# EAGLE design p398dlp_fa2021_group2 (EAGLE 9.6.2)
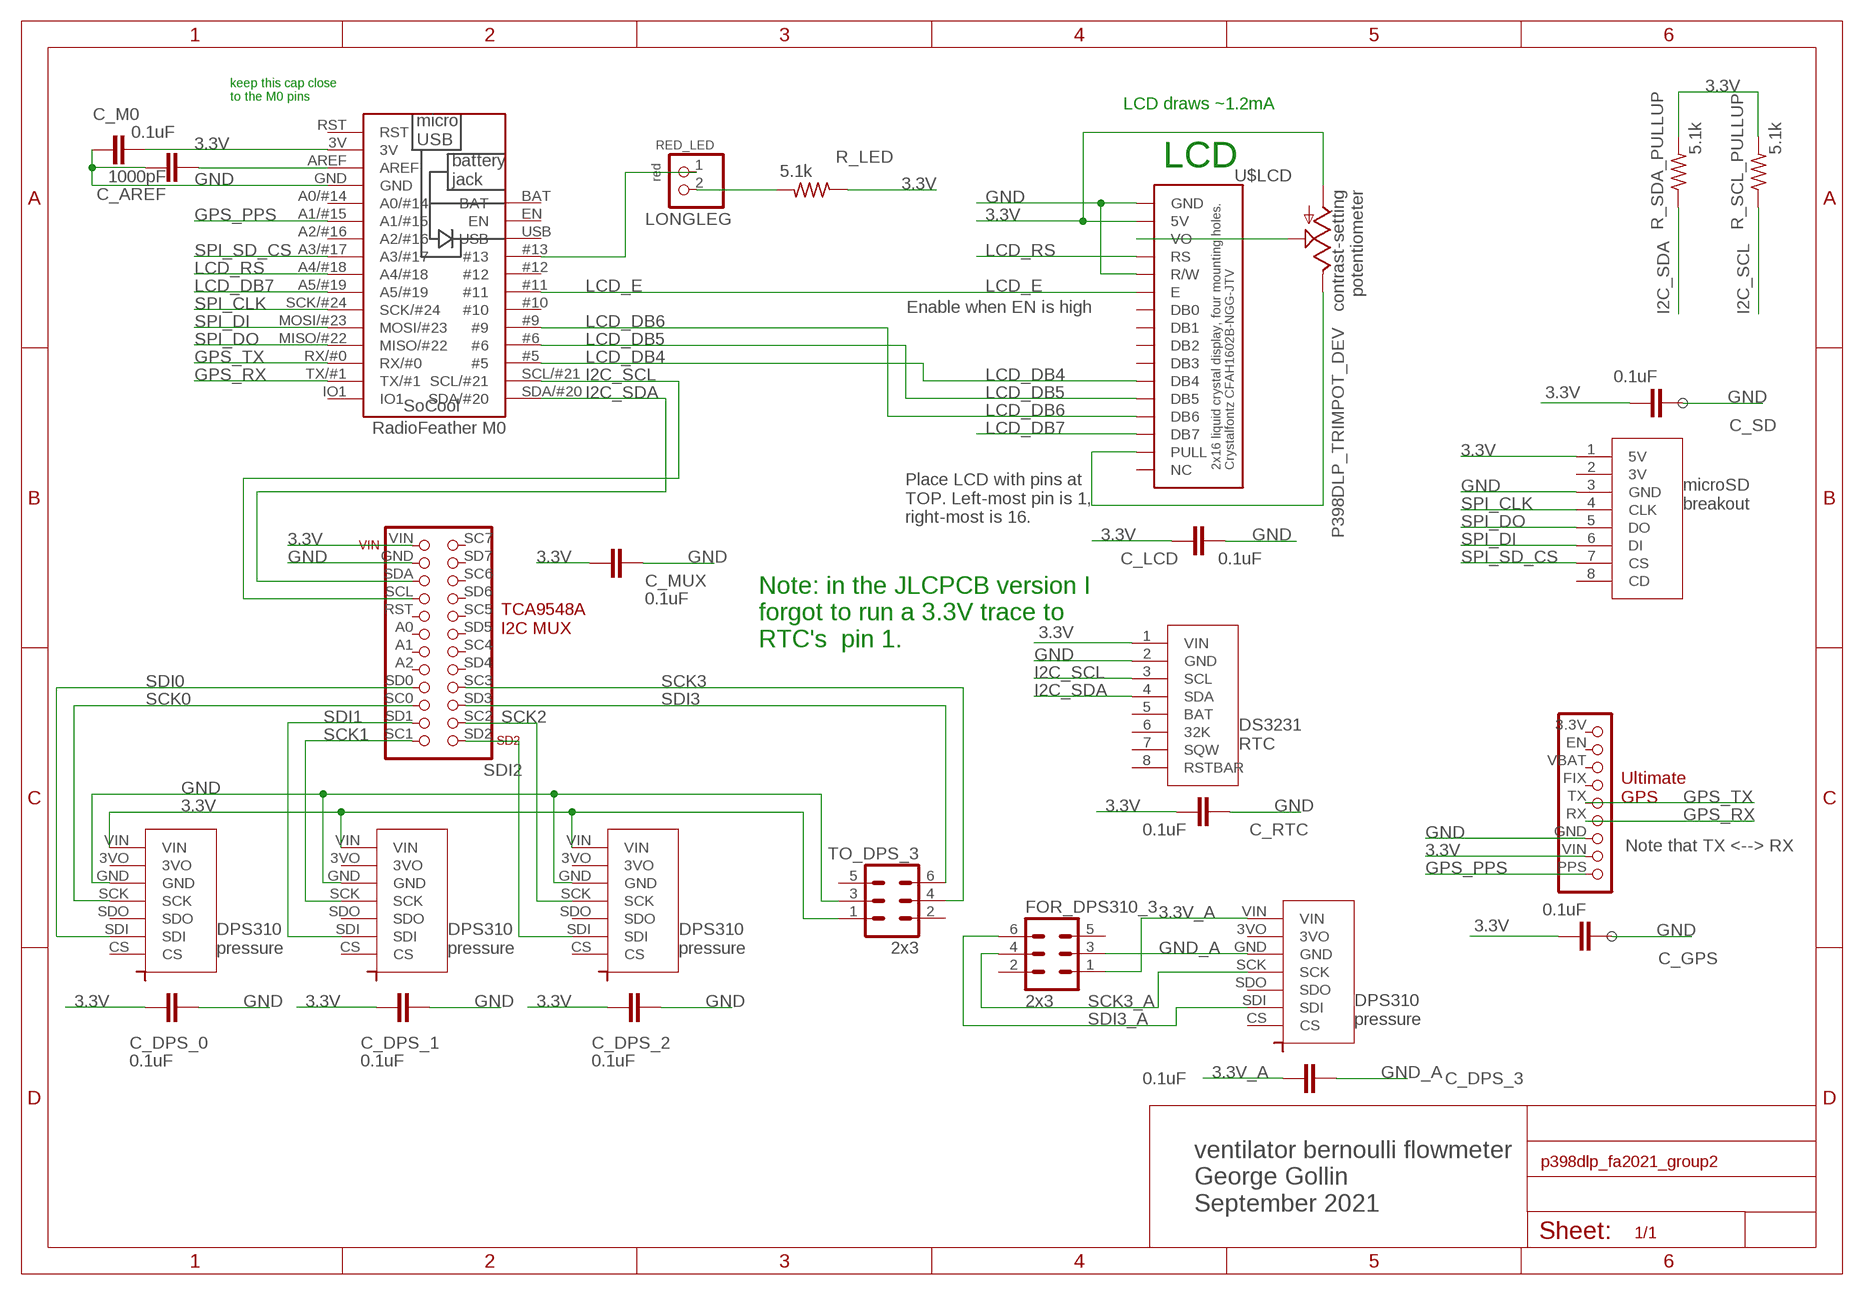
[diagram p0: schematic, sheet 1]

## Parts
C_AREF  1000pF  C5/3.5  [C5B3.5]
C_DPS_0  0.1uF  C5/3.5  [C5B3.5]
C_DPS_1  0.1uF  C5/3.5  [C5B3.5]
C_DPS_2  0.1uF  C5/3.5  [C5B3.5]
C_DPS_3  0.1uF  C5/3.5  [C5B3.5]
C_GPS  0.1uF  C5/3.5  [C5B3.5]
C_LCD  0.1uF  C5/3.5  [C5B3.5]
C_M0  0.1uF  C5/3.5  [C5B3.5]
C_MUX  0.1uF  C5/3.5  [C5B3.5]
C_RTC  0.1uF  C5/3.5  [C5B3.5]
C_SD  0.1uF  C5/3.5  [C5B3.5]
DPS310_0  P398DLP_DPS310_DEV  [P398DLP_DPS310_PKG]
DPS310_1  P398DLP_DPS310_DEV  [P398DLP_DPS310_PKG]
DPS310_2  P398DLP_DPS310_DEV  [P398DLP_DPS310_PKG]
DPS310_3  P398DLP_DPS310_DEV  [P398DLP_DPS310_PKG]
FOR_DPS310_3  2x3  P398DLP_RIBBON_PCB_2X3_DEV  [06V]
R_LED  5.1k  R-US_0207/7  [0207/7]
R_SCL_PULLUP  5.1k  R-US_0207/7  [0207/7]
R_SDA_PULLUP  5.1k  R-US_0207/7  [0207/7]
RED_LED  red  PINHD-1X2  [1X02]
TO_DPS_3  2x3  P398DLP_RIBBON_PCB_2X3_DEV  [06V]
U$5  P398DLP_TCA9548A_MUX_DEV  [P398DLP_TCA9548A_MUX_PKG]
U$6  P398DLP_DS3231_DEV  [P398DLP_DS3231_PKG]
U$19  P398DLP_TRIMPOT_DEV  [P398DLP_TRIMPOT_PKG]
U$GPS1  P398DLP_ULTIMATE_GPS_DEV  [P398DLP_ULTIMATE_GPS_PKG]
U$LCD  P398DLP_LCD_16X2_DEV  [P398DLP_LCD_16X2_PKG]
U$MICROSD1  P398DLP_MICROSD_DEV  [P398DLP_MICROSD_PKG]
U$RADIOFEATHER  P398DLP_RADIOFEATHER_MO_DEV  [P398DLP_RADIOFEATHER_M0_PKG]

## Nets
3.3V [power]: C_DPS_0.2 C_DPS_1.2 C_DPS_2.2 C_GPS.2 C_LCD.2 C_M0.1 C_MUX.2 C_RTC.2 C_SD.2 DPS310_0.VIN DPS310_1.VIN DPS310_2.VIN R_LED.1 R_SCL_PULLUP.2 R_SDA_PULLUP.2 TO_DPS_3.1 U$5.VIN U$6.1(VIN) U$19.BOTTOM U$GPS1.VIN U$LCD.5V U$MICROSD1.1(5V) U$RADIOFEATHER.3V
3.3V_A: C_DPS_3.2 DPS310_3.VIN FOR_DPS310_3.1
GND [power]: C_AREF.2 C_DPS_0.1 C_DPS_1.1 C_DPS_2.1 C_GPS.1 C_LCD.1 C_M0.2 C_MUX.1 C_RTC.1 C_SD.1 DPS310_0.GND DPS310_1.GND DPS310_2.GND TO_DPS_3.3 U$5.GND U$6.2(GND) U$GPS1.GND U$LCD.GND U$LCD.R/W U$MICROSD1.3(GND) U$RADIOFEATHER.GND
GND_A: C_DPS_3.1 DPS310_3.GND FOR_DPS310_3.3
GPS_PPS: U$GPS1.PPS U$RADIOFEATHER.A1/#15
GPS_RX: U$GPS1.RX U$RADIOFEATHER.TX/#1
GPS_TX: U$GPS1.TX U$RADIOFEATHER.RX/#0
I2C_SCL: R_SCL_PULLUP.1 U$5.SCL U$6.3(SCL) U$RADIOFEATHER.SCL/#21
I2C_SDA: R_SDA_PULLUP.1 U$5.SDA U$6.4(SDA) U$RADIOFEATHER.SDA/#20
LCD_DB4: U$LCD.DB4 U$RADIOFEATHER.#5
LCD_DB5: U$LCD.DB5 U$RADIOFEATHER.#6
LCD_DB6: U$LCD.DB6 U$RADIOFEATHER.#9
LCD_DB7: U$LCD.DB7 U$RADIOFEATHER.A5/#19
LCD_E: U$LCD.E U$RADIOFEATHER.#11
LCD_RS: U$LCD.RS U$RADIOFEATHER.A4/#18
LONGLEG: R_LED.2 RED_LED.2
N$1: U$19.TOP U$LCD.PULL
N$5: C_AREF.1 U$RADIOFEATHER.AREF
N$6: U$19.TAP U$LCD.VO
SCK0: DPS310_0.SCK U$5.SC0
SCK1: DPS310_1.SCK U$5.SC1
SCK2: DPS310_2.SCK U$5.SC2
SCK3: TO_DPS_3.4 U$5.SC3
SCK3_A: DPS310_3.SCK FOR_DPS310_3.4
SDI0: DPS310_0.SDI U$5.SD0
SDI1: DPS310_1.SDI U$5.SD1
SDI2: DPS310_2.SDI U$5.SD2
SDI3: TO_DPS_3.6 U$5.SD3
SDI3_A: DPS310_3.SDI FOR_DPS310_3.6
SPI_CLK: U$MICROSD1.4(CLK) U$RADIOFEATHER.SCK/#24
SPI_DI: U$MICROSD1.6(DI) U$RADIOFEATHER.MOSI/#23
SPI_DO: U$MICROSD1.5(DO) U$RADIOFEATHER.MISO/#22
SPI_SD_CS: U$MICROSD1.7(CS) U$RADIOFEATHER.A3/#17
WATCHDOG_PULSE: RED_LED.1 U$RADIOFEATHER.#13
Unconnected: DPS310_0.3VO DPS310_0.CS DPS310_0.SDO DPS310_1.3VO DPS310_1.CS DPS310_1.SDO DPS310_2.3VO DPS310_2.CS DPS310_2.SDO DPS310_3.3VO DPS310_3.CS DPS310_3.SDO FOR_DPS310_3.2 FOR_DPS310_3.5 TO_DPS_3.2 TO_DPS_3.5 U$5.A0 U$5.A1 U$5.A2 U$5.RST U$5.SC4 U$5.SC5 U$5.SC6 U$5.SC7 U$5.SD4 U$5.SD5 U$5.SD6 U$5.SD7 U$6.5(BAT) U$6.6(32K) U$6.7(SQW) U$6.8(RSTBAR) U$GPS1.3.3V U$GPS1.EN U$GPS1.FIX U$GPS1.VBAT U$LCD.DB0 U$LCD.DB1 U$LCD.DB2 U$LCD.DB3 U$LCD.NC U$MICROSD1.2(3V) U$MICROSD1.8(CD) U$RADIOFEATHER.#10 U$RADIOFEATHER.#12 U$RADIOFEATHER.A0/#14 U$RADIOFEATHER.A2/#16 U$RADIOFEATHER.BAT U$RADIOFEATHER.EN U$RADIOFEATHER.IO1 U$RADIOFEATHER.RST U$RADIOFEATHER.USB

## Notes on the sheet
- keep this cap close 
  to the M0 pins
- LCD draws ~1.2mA
- LCD
- contrast-setting
  potentiometer
- Enable when EN is high
- Place LCD with pins at 
  TOP. Left-most pin is 1, 
  right-most is 16.
- Note: in the JLCPCB version I
  forgot to run a 3.3V trace to
  RTC's  pin 1.
- Note that TX <--> RX
- ventilator bernoulli flowmeter
  George Gollin
  September 2021

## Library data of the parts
C_AREF C_DPS_0 C_DPS_1-C_DPS_3 C_GPS C_LCD C_M0 C_MUX C_RTC C_SD = capacitor-wima:C: CAPACITOR
DPS310_0 DPS310_1-DPS310_3 = p398dlp:P398DLP_DPS310_DEV: DPS310 precision pressure and temperature sensor. Adafruit 4494
FOR_DPS310_3 TO_DPS_3 = p398dlp:P398DLP_RIBBON_PCB_2X3_DEV: CONNECTOR; OC_FARNELL: unknown; OC_NEWARK: unknown
R_LED R_SCL_PULLUP R_SDA_PULLUP = resistor:R-US_: RESISTOR, American symbol
RED_LED = p398dlp_sp2020:PINHD-1X2: PIN HEADER
U$5 = p398dlp:P398DLP_TCA9548A_MUX_DEV: TCA9548A I2C MUX
U$6 = p398dlp:P398DLP_DS3231_DEV: DS3231 real time clock with battery backup
U$19 = p398dlp:P398DLP_TRIMPOT_DEV: trimpot
U$GPS1 = p398dlp:P398DLP_ULTIMATE_GPS_DEV: Adafruit "ultimate GPS" breakout board
U$LCD = p398dlp:P398DLP_LCD_16X2_DEV: 2x16 liquid crystal display, four mounting holes. Crystalfontz CFAH1602B-NGG-JTV
U$MICROSD1 = p398dlp:P398DLP_MICROSD_DEV: Adafruit microSD reader breakout board
U$RADIOFEATHER = p398dlp:P398DLP_RADIOFEATHER_MO_DEV: Adafruit RadioFeather M0 processor

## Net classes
1 power: width 0.305 mm

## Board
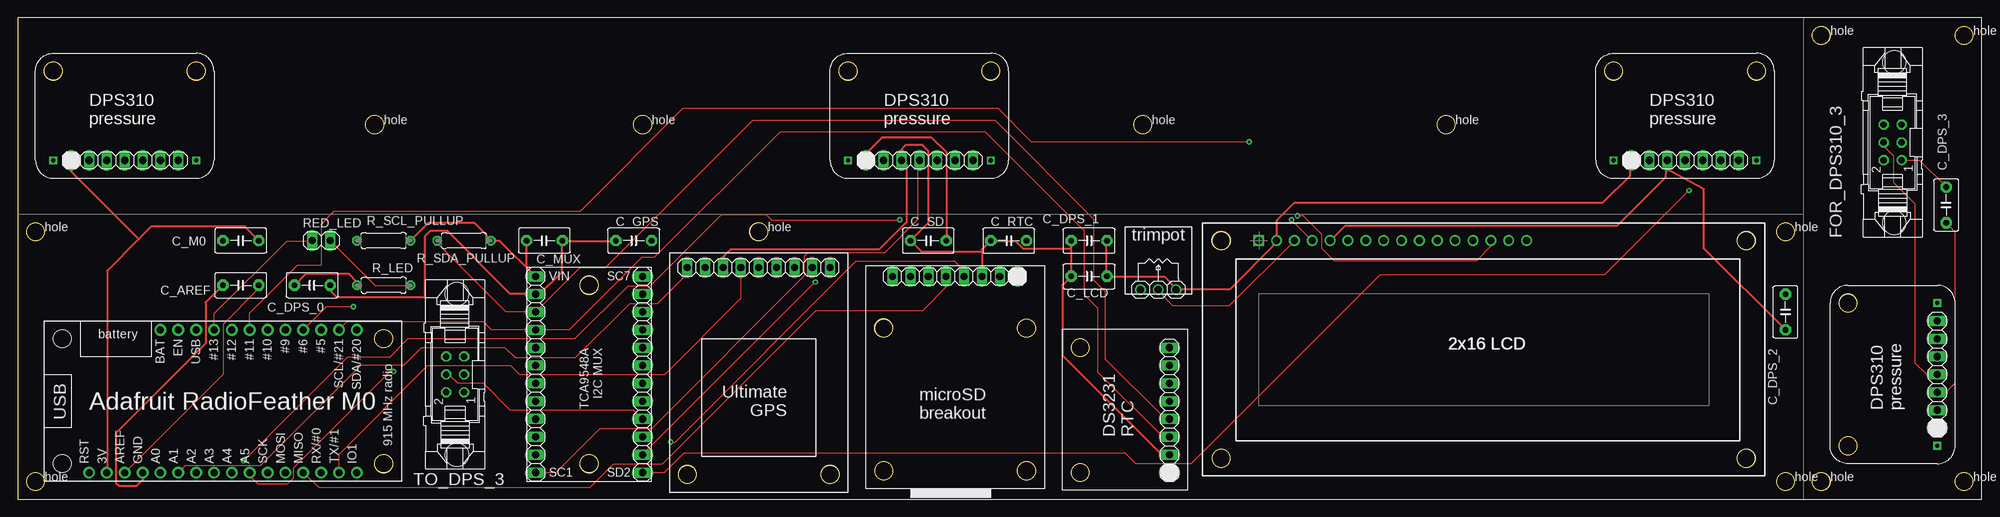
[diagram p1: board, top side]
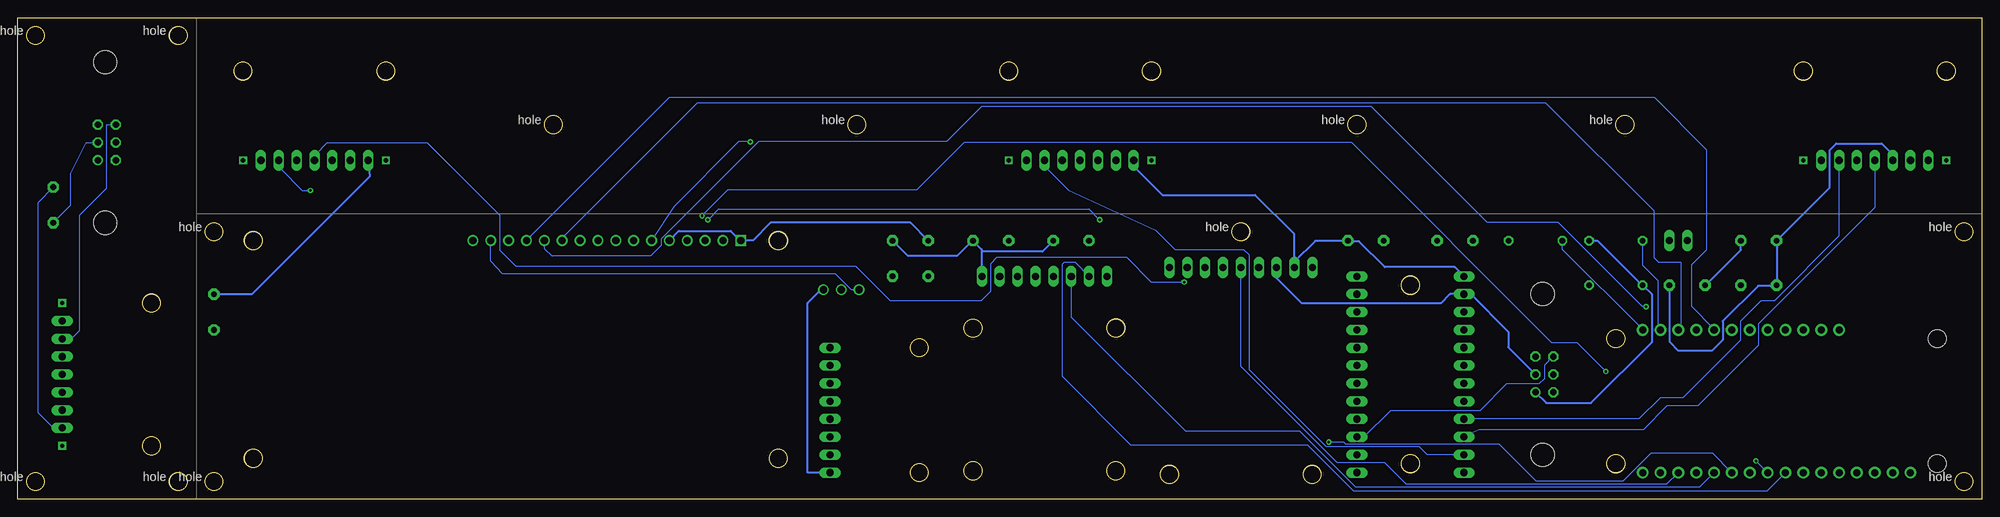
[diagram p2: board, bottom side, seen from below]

Size 279.4 x 68.58 mm. Coordinates in mm from the lower left corner, seen from the top.
Outline: 0,0 279.4,0 279.4,68.58 0,68.58 0,0
Copper layers (1*16): Top 0.035mm / dielectric 1.5mm / Bottom 0.035mm
Design rules "default": minimum track width 6mil, minimum drill 0.35mm, track to track 6mil, track to pad 6mil, pad to pad 6mil, via to via 6mil, smd to smd 6mil, copper to edge 40mil, drill to drill 6mil, minimum pad ring 10mil, minimum via ring 8mil, stop-mask expansion 4mil, vias tented up to drill 0mil, thermal gap 10mil

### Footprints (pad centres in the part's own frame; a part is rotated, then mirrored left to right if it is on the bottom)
C5B3.5 = drill 0.813 pad 1.6 octagon: 1 -2.54,0; 2 2.54,0
P398DLP_DPS310_PKG = drill 1.016 long: 3VO 7.62,2.54; CS 20.32,2.54; GND 10.16,2.54; SCK 12.7,2.54; SDI 17.78,2.54; SDO 15.24,2.54; VIN 5.08,2.54 | drill 0.6 square: P$1 2.54,2.54; P$2 22.86,2.54 | hole 2.54: 22.86,15.24; 2.54,15.24
06V = drill 0.914: 1 -2.54,-1.27 | drill 0.914 octagon: 2 -2.54,1.27; 3 0,-1.27; 4 0,1.27; 5 2.54,-1.27; 6 2.54,1.27 | hole 3.302: 11.43,-0.254; -11.43,-0.254
0207/7 = drill 0.813 octagon: 1 -3.81,0; 2 3.81,0
1X02 = drill 1.016 long: 1 -1.27,0; 2 1.27,0
P398DLP_MOUNTING_HOLE_PKG = hole 2.54: 0,0
P398DLP_TCA9548A_MUX_PKG = drill 1.016 long: A0 12.7,0; A1 15.24,0; A2 17.78,0; GND 2.54,0; RST 10.16,0; SC0 22.86,0; SC1 27.94,0; SC2 25.4,15.24; SC3 20.32,15.24; SC4 15.24,15.24; SC5 10.16,15.24; SC6 5.08,15.24; SC7 0,15.24; SCL 7.62,0; SD0 20.32,0; SD1 25.4,0; SD2 27.94,15.24; SD3 22.86,15.24; SD4 17.78,15.24; SD5 12.7,15.24; SD6 7.62,15.24; SD7 2.54,15.24; SDA 5.08,0; VIN 0,0 | hole 2.54: 1.27,7.62; 26.67,7.62
P398DLP_DS3231_PKG = drill 1.016 long: 1 0,0; 2 2.54,0; 3 5.08,0; 4 7.62,0; 5 10.16,0; 6 12.7,0; 7 15.24,0; 8 17.78,0 | hole 2.54: 0,12.7; 17.78,12.7
P398DLP_TRIMPOT_PKG = drill 1.016: BOTTOM 7.303,0.635; TAP 4.763,0.635; TOP 2.223,0.635
P398DLP_ULTIMATE_GPS_PKG = drill 1.016 long: 3.3V 0,0; EN 2.54,0; FIX 7.62,0; GND 15.24,0; PPS 20.32,0; RX 12.7,0; TX 10.16,0; VBAT 5.08,0; VIN 17.78,0 | hole 2.54: 0,29.464; 20.32,29.464
P398DLP_LCD_16X2_PKG = drill 1.016: 5V 2.544,0.006; DB0 15.244,0.006; DB1 17.784,0.006; DB2 20.324,0.006; DB3 22.864,0.006; DB4 25.404,0.006; DB5 27.944,0.006; DB6 30.484,0.006; DB7 33.024,0.006; E 12.704,0.006; NC 38.104,0.006; PULL 35.564,0.006; R/W 10.164,0.006; RS 7.624,0.006; VO 5.084,0.006 | drill 1.016 square: GND 0.004,0.006 | hole 2.54: -5.334,0; -5.334,-30.988; 69.342,-30.988; 69.342,0
P398DLP_MICROSD_PKG = drill 1.016 long: 1 0,0; 2 2.54,0; 3 5.08,0; 4 7.62,0; 5 10.16,0; 6 12.7,0; 7 15.24,0; 8 17.78,0 | hole 2.54: -1.27,27.686; 19.05,27.686; 19.05,7.366; -1.27,7.366
P398DLP_RADIOFEATHER_M0_PKG = drill 1 pad 1.676: 3V 8.89,1.27; #5 39.37,21.59; #6 36.83,21.59; #9 34.29,21.59; #10 31.75,21.59; #11 29.21,21.59; #12 26.67,21.59; #13 24.13,21.59; A0/#14 16.51,1.27; A1/#15 19.05,1.27; A2/#16 21.59,1.27; A3/#17 24.13,1.27; A4/#18 26.67,1.27; A5/#19 29.21,1.27; AREF 11.43,1.27; BAT 16.51,21.59; EN 19.05,21.59; GND 13.97,1.27; IO1 44.45,1.27; MISO/#22 36.83,1.27; MOSI/#23 34.29,1.27; RST 6.35,1.27; RX/#0 39.37,1.27; SCK/#24 31.75,1.27; SCL/#21 41.91,21.59; SDA/#20 44.45,21.59; TX/#1 41.91,1.27; USB 21.59,21.59 | hole 2.54: 48.26,2.54; 48.26,20.32; 2.54,20.32; 2.54,2.54

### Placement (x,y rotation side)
C_AREF  31.75,30.48 180 top
C_DPS_0  41.91,30.48 180 top
C_DPS_1  152.4,36.83 0 top
C_DPS_2  251.46,26.67 90 top
C_DPS_3  274.32,41.91 90 top
C_GPS  87.63,36.83 0 top
C_LCD  152.4,31.75 0 top
C_M0  31.75,36.83 180 top
C_MUX  74.93,36.83 180 top
C_RTC  140.97,36.83 0 top
C_SD  129.54,36.83 0 top
DPS310_0  2.54,45.72 0 top
DPS310_1  115.57,45.72 0 top
DPS310_2  224.47,45.72 0 top
DPS310_3  275.59,5.08 90 top
FOR_DPS310_3  266.7,50.8 90 top
R_LED  52.07,30.48 0 top
R_SCL_PULLUP  52.07,36.83 0 top
R_SDA_PULLUP  63.5,36.83 0 top
RED_LED  43.18,36.83 0 top
TO_DPS_3  62.23,17.78 90 top
U$1  [P398DLP_MOUNTING_HOLE_PKG]  2.54,2.54 0 top
U$2  [P398DLP_MOUNTING_HOLE_PKG]  2.54,38.1 0 top
U$3  [P398DLP_MOUNTING_HOLE_PKG]  105.41,38.1 0 top
U$4  [P398DLP_MOUNTING_HOLE_PKG]  251.46,2.54 0 top
U$5  73.66,31.75 270 top
U$6  163.83,3.81 90 top
U$7  [P398DLP_MOUNTING_HOLE_PKG]  251.46,38.1 0 top
U$8  [P398DLP_MOUNTING_HOLE_PKG]  256.54,66.04 0 top
U$9  [P398DLP_MOUNTING_HOLE_PKG]  276.86,66.04 0 top
U$10  [P398DLP_MOUNTING_HOLE_PKG]  256.54,2.54 0 top
U$11  [P398DLP_MOUNTING_HOLE_PKG]  276.86,2.54 0 top
U$12  [P398DLP_MOUNTING_HOLE_PKG]  50.8,53.34 0 top
U$13  [P398DLP_MOUNTING_HOLE_PKG]  88.9,53.34 0 top
U$14  [P398DLP_MOUNTING_HOLE_PKG]  160.02,53.34 0 top
U$15  [P398DLP_MOUNTING_HOLE_PKG]  203.2,53.34 0 top
U$19  157.48,29.21 0 top
U$GPS1  115.57,33.02 180 top
U$LCD  176.53,36.83 0 top
U$MICROSD1  142.24,31.75 180 top
U$RADIOFEATHER  3.81,2.54 0 top

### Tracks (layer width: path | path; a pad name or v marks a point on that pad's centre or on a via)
3.3V
  Top 0.305: DPS310_0.VIN 7.62,46.69 17.25,37.06 | C_M0.1 34.29,36.88 32.33,38.84 19.02,38.84 17.25,37.06 | 17.25,37.06 12.72,32.54 12.72,3.81 U$RADIOFEATHER.3V | R_LED.1 48.26,30.94 47.07,32.13 41.05,32.13 39.4,30.48 C_DPS_0.2 | R_SCL_PULLUP.2 58.45,39.4 64.92,39.4 67.31,37.01 R_SDA_PULLUP.2 67.36,36.8 68.58,36.8 73.61,31.77 U$5.VIN 72.39,33.02 C_MUX.2 | C_DPS_1.2 154.91,36.8 154.91,31.85 C_LCD.2 154.99,31.7 163.09,31.7 164.78,30.01 U$19.BOTTOM 164.9,29.95 172.49,29.95 179.07,36.53 U$LCD.5V 179.15,36.96 179.15,39.73 181.63,42.22 225.48,42.22 229.36,46.1 229.36,48.23 DPS310_2.VIN | DPS310_1.VIN 120.4,48.9 122.99,51.49 130.02,51.49 132.1,49.4 132.1,36.85 C_SD.2
  Bottom 0.305: R_SCL_PULLUP.2 55.85,36.8 54.63,36.8 48.31,30.48 R_LED.1 48.16,30.4 46.97,29.21 46.97,22.35 55.6,13.72 61.98,13.72 TO_DPS_3.1 | U$5.VIN 74.98,33.07 84.94,33.07 88.59,36.73 90.07,36.73 C_GPS.2 90.22,36.8 94.82,36.8 97.79,33.83 U$GPS1.VIN 97.79,37.74 103.38,43.33 116.56,43.33 120.4,47.17 120.4,48.23 DPS310_1.VIN | C_M0.1 34.29,35.51 39.32,30.48 C_DPS_0.2 | DPS310_2.VIN 229.34,45.95 246.02,29.26 251.46,29.26 C_DPS_2.2 | 142.26,35.28 142.26,35.59 C_RTC.2 143.64,36.8 145.8,34.65 152.76,34.65 C_DPS_1.2 | 142.26,35.28 142.26,31.77 U$MICROSD1.1 | 142.26,35.28 133.66,35.28 132.13,36.8 C_SD.2 | U$6.1 167,3.81 167,27.94 165.1,29.84 U$19.BOTTOM
3.3V_A
  Top 0.152: FOR_DPS310_3.1 268,48.23 270.59,48.23 274.32,44.5 C_DPS_3.2
  Bottom 0.152: DPS310_3.VIN 274.32,10.16 276.56,12.39 276.56,42.19 274.32,44.42 C_DPS_3.2
GND
  Top 0.305: U$RADIOFEATHER.GND 17.78,2.77 16.92,1.91 14.45,1.91 13.97,2.39 13.97,9.42 26.75,22.2 26.75,28.04 29.18,30.48 C_AREF.2 | 77.42,36.8 77.42,32.36 74.27,29.21 U$5.GND 73.53,29.26 70.05,29.26 61.14,38.18 58.65,38.18 57.91,37.44 57.91,28.8 57.84,28.73 45.47,28.73 44.45,29.74 C_DPS_0.1 | 77.42,36.8 77.42,36.83 C_MUX.1 | 77.42,36.8 85.04,36.8 C_GPS.1 | C_DPS_2.1 251.46,24.16 239.88,35.74 239.88,44.17 234.42,47.1 DPS310_2.GND 234.42,45.85 227.53,38.96 188.85,38.96 186.77,36.88 U$LCD.R/W | 137.16,35.28 137.16,35.59 138.38,36.8 C_RTC.1 138.53,36.73 142.04,36.73 143.1,35.66 149.88,35.66 | 137.16,35.28 U$MICROSD1.3 | 127.03,36.88 129.54,39.4 129.54,49.58 128.73,50.39 126.29,50.39 125.48,49.59 DPS310_1.GND 125.81,48.23 126.44,47.6 126.44,39.47 122.56,35.59 101.45,35.59 100.33,34.47 U$GPS1.GND | 127.03,36.88 126.99,36.84 128.55,35.28 137.16,35.28 | 127.03,36.88 C_SD.1 | U$6.2 163.83,6.4 162.69,6.4 148.59,20.5 148.59,30.48 C_LCD.1 149.88,31.85 149.88,35.66 | 149.88,35.66 149.88,36.8 C_DPS_1.1
  Bottom 0.305: DPS310_0.GND 12.7,49.07 14.28,50.65 20.73,50.65 21.67,49.71 21.67,44.4 29.18,36.88 C_M0.2 29.18,36.73 29.18,30.48 C_AREF.2 29.34,30.4 31.83,30.4 36.85,25.38 36.85,22.71 38.41,21.16 43.16,21.16 44.42,22.43 44.42,30.48 C_DPS_0.1 | TO_DPS_3.3 67.36,21.64 67.36,23.85 72.72,29.21 U$5.GND 75.64,29.21 76.96,27.89 96.72,27.89 100.33,31.5 U$GPS1.GND | U$LCD.R/W 186.69,36.88 185.37,38.2 177.98,38.2 176.66,36.88 176.56,36.88 U$LCD.GND 176.4,36.88 174.8,36.88 172.29,39.4 152.4,39.4 149.88,36.88 C_DPS_1.1
GND_A
  Top 0.152: DPS310_3.GND 274.24,15.24 275.54,16.54 275.54,38.1 274.32,39.32 C_DPS_3.1
  Bottom 0.152: FOR_DPS310_3.3 269.65,50.8 271.86,46.38 271.86,41.86 274.32,39.4 C_DPS_3.1
GPS_PPS
  Top 0.152: U$GPS1.PPS 95.25,32.11 91.06,27.91 87.1,27.91 79.38,20.19 70.74,20.19 69.28,21.65 57.47,21.65 54.99,19.18 48.9,19.18 34.59,4.88 23.93,4.88 U$RADIOFEATHER.A1/#15
GPS_RX
  Top 0.152: U$GPS1.RX 102.87,28.57 92.08,17.78 71.37,17.78 70.1,19.05 58.34,19.05 45.72,6.43 U$RADIOFEATHER.TX/#1
GPS_TX
  Bottom 0.152: U$GPS1.TX 105.39,32.99 105.39,18.9 91.67,5.18 84.89,5.18 81.86,2.16 44.86,2.16 43.2,3.81 U$RADIOFEATHER.RX/#0
I2C_SCL
  Top 0.152: U$RADIOFEATHER.SCL/#21 45.72,24.16 46.86,25.3 66.19,25.3 67.33,24.16 73.61,24.16 U$5.SCL 73.69,24.16 78.49,24.16 88.82,34.49 90.63,34.49 108.51,52.38 137.59,52.38 151.71,38.25 151.71,29.18 153.62,27.28 153.62,18.16 162.89,8.89 U$6.3
  Bottom 0.152: U$RADIOFEATHER.SCL/#21 46.1,24.51 46.1,31.17 48.23,33.3 48.23,36.8 R_SCL_PULLUP.1
I2C_SDA
  Top 0.152: U$6.4 163.25,11.43 154.69,19.99 154.69,29.59 153.03,31.24 153.03,39.93 139.01,53.95 104.6,53.95 83.64,32.99 80.01,32.99 73.69,26.67 U$5.SDA 69.49,26.67 59.69,36.47 R_SDA_PULLUP.1
  Bottom 0.152: R_SDA_PULLUP.1 59.66,36.8 59.66,35.59 48.23,24.16 U$RADIOFEATHER.SDA/#20
LCD_DB4
  Bottom 0.152: U$RADIOFEATHER.#5 42.82,24.49 42.82,33.71 45.97,33.71 46.61,34.34 46.61,41.02 62,56.41 182.78,56.41 202.18,37.01 201.92,37.01 U$LCD.DB4
LCD_DB5  (via drill 0.35)
  Top 0.152: v47.78,27.43 43.97,27.43 40.69,24.16 U$RADIOFEATHER.#6
  Bottom 0.152: U$LCD.DB5 204.47,35.74 203.4,34.67 189.33,34.67 187.88,36.12 187.88,37.06 174.04,50.9 147.27,50.9 142.29,55.88 86.84,55.88 70.36,39.4 60.25,39.4 48.28,27.43 v47.78,27.43
LCD_DB6
  Bottom 0.152: U$LCD.DB6 206.65,37.13 206.78,37.13 186.77,57.15 46.56,57.15 39.12,49.71 39.12,35.56 41.26,33.41 41.26,27.45 38.1,24.28 U$RADIOFEATHER.#9
LCD_DB7  (via drill 0.35)
  Top 0.152: U$LCD.DB7 209.55,36.05 207.54,34.04 187.2,34.04 185.42,35.81 185.42,37.77 182.8,40.39 v182.04,40.39 | v53.49,18.21 52.98,18.21 39.29,4.52 39.29,3.1 38.43,2.23 34.14,2.23 33.02,3.35 U$RADIOFEATHER.A5/#19
  Bottom 0.152: v182.04,40.39 178.36,44.07 151.49,44.07 144.81,50.75 89.61,50.75 61.14,22.28 57.56,22.28 v53.49,18.21
LCD_E  (via drill 0.35)
  Top 0.152: v175.18,50.9 144.17,50.9 139.42,55.65 94.67,55.65 80.06,41.05 45.06,41.05 43.16,39.14 43.16,35.94 43.16,33.3 43.18,33.27 39.75,33.27 33.02,26.54 U$RADIOFEATHER.#11
  Bottom 0.152: v175.18,50.9 176.84,50.9 186.05,41.68 U$LCD.E
LCD_RS  (via drill 0.35)
  Top 0.152: v181.2,39.78 184.1,36.88 U$LCD.RS | v125.5,39.78 107.21,39.78 106.45,40.54 100.15,40.54 89.99,30.38 86.82,30.38 79.32,22.89 55.58,22.89 52.91,20.22 46.89,20.22 v32.16,5.49
  Bottom 0.152: v125.5,39.78 127.03,41.3 179.68,41.3 v181.2,39.78 | U$RADIOFEATHER.A4/#18 v32.16,5.49
LONGLEG
  Top 0.152: R_LED.2 50.83,30.48 44.5,36.8 RED_LED.2
N$1
  Bottom 0.152: U$19.TOP 159.72,29.87 160.86,29.87 163.14,32.16 210.46,32.16 212.09,33.9 U$LCD.PULL
N$5
  Top 0.152: C_AREF.1 34.29,30 29.29,24.99 29.29,17.86 U$RADIOFEATHER.AREF
N$6
  Top 0.152: U$19.TAP 162.24,29.65 164.36,27.53 172.31,27.53 181.59,36.8 U$LCD.VO
SCK0
  Bottom 0.152: DPS310_0.SCK 15.24,41.5 31.8,24.94 31.8,21.92 40.44,13.28 44.81,13.28 48.16,9.93 71.58,9.93 U$5.SC0
SCK1
  Top 0.152: U$5.SC1 76.5,3.81 82.75,10.06 90.14,10.06 111.89,31.8 111.89,34.59 112.37,35.08 123.29,35.08 128.02,39.8 128.02,48.23 DPS310_1.SCK
SCK2  (via drill 0.35)
  Top 0.152: v113.46,30.94 88.92,6.4 U$5.SC2
  Bottom 0.152: v113.46,30.94 118.16,30.94 121.69,34.47 140.08,34.47 140.94,33.6 140.94,29.67 142.32,28.3 155.3,28.3 160.22,33.22 208.56,33.22 210.82,35.48 210.82,40.44 221.13,50.75 235.36,50.75 236.96,49.15 DPS310_2.SCK
SCK3
  Top 0.152: TO_DPS_3.4 60.96,17.75 61.42,17.75 62.69,16.48 66.27,16.48 70.08,12.68 87.61,12.68 88.85,11.43 U$5.SC3
SCK3_A
  Top 0.152: DPS310_3.SCK 271.55,17.78 269.95,19.38 269.95,42.04 266.88,45.11 266.88,48.84 265.48,50.24 265.48,50.75 FOR_DPS310_3.4
SDI0
  Bottom 0.152: U$5.SD0 48.77,11.43 45.72,14.48 42.52,14.48 34.39,22.61 34.39,25.3 31.42,28.27 29.57,28.27 20.34,37.49 20.34,48.23 DPS310_0.SDI
SDI1
  Bottom 0.152: U$5.SD1 73.69,6.4 78.97,6.4 80.11,7.54 93.32,7.54 104.27,18.49 104.27,34.85 105,35.59 114.81,35.59 117.54,38.32 129.91,44.05 133.1,47.24 DPS310_1.SDI
SDI2  (via drill 0.35)
  Top 0.152: U$5.SD2 91.97,3.81 94.72,6.55 157.58,6.55 159.06,5.08 166.93,5.08 193.8,31.95 225.73,31.95 v237.74,43.97
  Bottom 0.152: DPS310_2.SDI 242.04,47.12 238.89,43.97 v237.74,43.97
SDI3
  Bottom 0.152: TO_DPS_3.6 61.04,20.32 62.18,19.18 62.18,17.25 62.94,16.48 67.54,16.48 71.35,12.68 84.1,12.68 87.88,8.89 U$5.SD3
SDI3_A
  Bottom 0.152: FOR_DPS310_3.6 266.75,53.34 266.75,44.3 270.59,40.46 270.59,24.03 271.75,22.86 DPS310_3.SDI
SPI_CLK  (via drill 0.35)
  Top 0.152: U$MICROSD1.4 134.62,32.56 133.27,33.91 119.28,33.91 93.52,8.15 v92.89,8.15
  Bottom 0.152: v92.89,8.15 90.75,8.15 90.45,7.85 68.66,7.85 63.4,2.59 51.05,2.59 47.12,6.53 38.3,6.53 35.59,3.81 U$RADIOFEATHER.SCK/#24
SPI_DI
  Bottom 0.152: U$MICROSD1.6 129.54,25.98 113.23,9.68 97,9.68 89.05,1.73 40.18,1.73 U$RADIOFEATHER.MOSI/#23
SPI_DO
  Top 0.152: U$MICROSD1.5 132.08,30.2 128.78,26.9 113.56,26.9 91.72,5.05 84.76,5.05 81.41,1.7 42.8,1.7 40.69,3.81 U$RADIOFEATHER.MISO/#22
SPI_SD_CS
  Bottom 0.152: U$MICROSD1.7 129.03,33.78 130.5,33.78 130.78,33.5 130.78,17.48 121.03,7.72 95.89,7.72 89.33,1.17 30.61,1.17 27.96,3.81 U$RADIOFEATHER.A3/#17
WATCHDOG_PULSE
  Top 0.152: RED_LED.1 41.91,36.8 38.33,36.8 27.96,26.44 27.96,24.16 U$RADIOFEATHER.#13

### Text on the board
tDocu: JLCJLCJLCJLC | George Gollin, University of Illinois / p398dlp_fa2021_ventilator / Fille de Lear Designs / September 2021 | long leg
bDocu: George Gollin, University of Illinois / p398dlp_fa2021_ventilator / Fille de Lear Designs / September 2021 | George Gollin, University of Illinois / p398dlp_fa2021_ventilator / Fille de Lear Designs / September 2021 | George Gollin, University of Illinois / p398dlp_fa2021_ventilator / Fille de Lear Designs / September 2021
